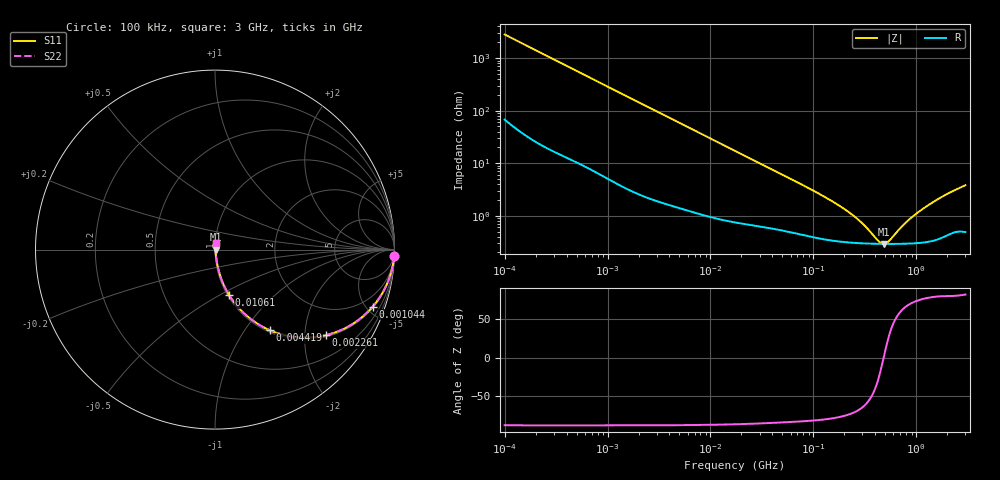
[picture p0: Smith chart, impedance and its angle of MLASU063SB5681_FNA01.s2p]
! MLASU063SB5681_FNA01  S-PARAMETER MODEL  ( Standard Model )
! Model Generated by TAIYO YUDEN Corporation (http://www.ty-top.com)
! Version 1.0
! TAIYO YUDEN Control No. 220601
! Copyright(c) 2012 TAIYO YUDEN CO.,LTD. All Rights Reserved.
! Product Description (link to TY-COMPAS)
! https://ds.yuden.co.jp/TYCOMPAS/or/detail?pn=MLASU063SB5681KFNA01&u=M
! Products Name : Multilayer Ceramic Capacitors
! Characteristics :
!  Capacitance : 680 [pF] , Rated Voltage : 50 [V] , TCC : B / X5R
!  Case Size : 0.6 x 0.3 / 0.024 x 0.012 [mm/inch] , Thickness : 0.3 / 0.012 [mm/inch]
!  (Conditions: Temperature = 25 [degC] , DC Bias Voltage = 0 [V])
! External Node Assignments :
!  1  o---| |---o  2
! GND o---------o GND
! Frequency Range : 100kHz  -  3GHz  [ 401 STEP ]
# MHZ S RI R 50
! Freq[MHz].  S11 Real  S11 Imag  S21 Real  S21 Imag  S12 Real  S12 Imag  S22 Real  S22 Imag
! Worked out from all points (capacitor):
!   401 points, 100 kHz to 3 GHz, reference 50 ohm
!   read as one part in series: C = 564 pF near 105.3 kHz
!   lowest |Z| = 291 mohm at 481.3 MHz (marker M1)
!   series resonance near 481.9 MHz, so ESL is about 190 pH
!   S11 on the Smith chart (normalised r, x): 100 kHz: 2, -56; 1.044 MHz: 1.10, -5.51; 2.261 MHz: 1.05, -2.56; 4.419 MHz: 1.03, -1.32; 10.61 MHz: 1.02, -0.55; 3 GHz: 1.01, +0.08
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0.1  0.9979 -0.0354  0.0021 0.0354  0.0021 0.0354  0.9979 -0.0354
0.259498  0.9901 -0.0905  0.00988 0.0905  0.00988 0.0905  0.9901 -0.0905
0.562235  0.9595 -0.1882  0.0405 0.1882  0.0405 0.1882  0.9595 -0.1882
1.043626  0.8793 -0.3171  0.1207 0.3171  0.1207 0.3171  0.8793 -0.3171
1.536162  0.7752 -0.4089  0.2248 0.4089  0.2248 0.4089  0.7752 -0.4089
2.261149  0.6187 -0.4767  0.3813 0.4767  0.3813 0.4767  0.6187 -0.4767
3.161081  0.458 -0.4883  0.542 0.4883  0.542 0.4883  0.458 -0.4883
4.419184  0.3065 -0.4498  0.6935 0.4498  0.6935 0.4498  0.3065 -0.4498
6.674626  0.1675 -0.3603  0.8325 0.3603  0.8325 0.3603  0.1675 -0.3603
10.61445  0.0784 -0.2528  0.9216 0.2528  0.9216 0.2528  0.0784 -0.2528
17.7727  0.0336 -0.1594  0.9664 0.1594  0.9664 0.1594  0.0336 -0.1594
37.52708  0.012 -0.0782  0.988 0.0782  0.988 0.0782  0.012 -0.0782
97.38194  0.00484 -0.0304  0.9952 0.0304  0.9952 0.0304  0.00484 -0.0304
227.9507  0.00319 -0.0107  0.9968 0.0107  0.9968 0.0107  0.00319 -0.0107
302.6647  0.00301 -0.00629  0.997 0.00629  0.997 0.00629  0.00301 -0.00629
434.1712  0.00291 -0.00137  0.9971 0.00137  0.9971 0.00137  0.00291 -0.00137
481.3181  0.0029 -1.51e-05  0.9971 1.51e-05  0.9971 1.51e-05  0.0029 -1.51e-05
547.5153  0.0029 0.00168  0.9971 -0.00168  0.9971 -0.00168  0.0029 0.00168
785.4083  0.00297 0.00667  0.997 -0.00667  0.997 -0.00667  0.00297 0.00667
1097.999  0.00318 0.0121  0.9968 -0.0121  0.9968 -0.0121  0.00318 0.0121
1838.476  0.00445 0.0233  0.9955 -0.0233  0.9955 -0.0233  0.00445 0.0233
3000  0.00627 0.0374  0.9937 -0.0374  0.9937 -0.0374  0.00627 0.0374
